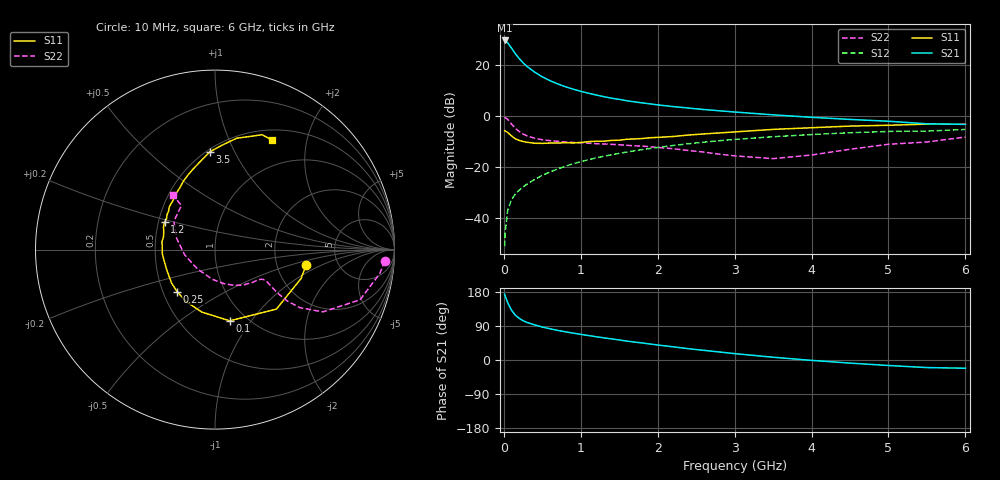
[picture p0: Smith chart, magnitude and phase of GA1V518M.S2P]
! Infineon Technologies  Discrete & RF Semiconductors
! BF775
! Si NPN RF Bipolar Junction Transistor in SOT23
! VCE = 1.5 V  IC = 18 mA
! Common Emitter S-Parameters:  May  1996
# GHz  S  MA  R  50
!  f  S11  S21  S12  S22
! GHz  MAG  ANG  MAG  ANG  MAG  ANG  MAG  ANG
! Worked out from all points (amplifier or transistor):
!   36 points, 10 MHz to 6 GHz, reference 50 ohm
!   highest |S21| = 29.6 dB at 10 MHz (marker M1)
!   |S21| within 3 dB of that: start of sweep to 99.22 MHz
!   unconditionally stable (mu >= 1): 326.7 MHz to end of sweep
!   at 250 MHz: K = 0.91, MSG = 24.3 dB, |S12| = -27.8 dB
!   at 1.4 GHz: K = 1.17, MAG = 8.6 dB, |S12| = -15.2 dB
!   at 6 GHz: K = 1.02, MAG = 0.2 dB, |S12| = -5.3 dB
!   S11 on the Smith chart (normalised r, x): 10 MHz: 2.94, -0.69; 100 MHz: 0.84, -0.79; 250 MHz: 0.59, -0.31; 1.2 GHz: 0.54, +0.18; 3.5 GHz: 0.52, +0.80; 6 GHz: 0.63, +1.45
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0.01  0.5145 -9.6  30.2 173.7  0.0028 81.6  0.9471 -3.9
0.02  0.5058 -18.6  29.73 167.5  0.0056 81.5  0.9282 -8.2
0.05  0.4765 -44.1  27.17 151.2  0.014 73.2  0.8551 -19.1
0.1  0.4052 -78.3  21.3 131.3  0.023 65.9  0.6941 -30.0
0.15  0.3557 -102.0  16.54 118.1  0.0296 62.8  0.5721 -34.4
0.2  0.3312 -119.1  13.34 109.9  0.0351 62.8  0.495 -35.4
0.25  0.3153 -132.2  11 103.7  0.0406 63.7  0.4423 -35.0
0.3  0.3053 -142.5  9.382 99.2  0.0459 64.8  0.4079 -34.3
0.4  0.2917 -157.1  7.23 92.6  0.0568 66.5  0.3666 -32.9
0.5  0.2901 -167.3  5.834 87.0  0.0683 67.7  0.3421 -31.8
0.6  0.2943 -175.6  4.913 82.4  0.0799 67.8  0.3279 -31.5
0.7  0.2944 177.4  4.25 78.1  0.0915 68.1  0.3182 -31.7
0.8  0.2985 171.5  3.739 74.5  0.1035 67.1  0.3091 -32.3
0.9  0.2955 165.8  3.352 70.9  0.1156 66.7  0.303 -33.1
1.1  0.3135 156.2  2.789 64.5  0.1385 65.4  0.2922 -35.9
1.2  0.3192 151.5  2.577 61.4  0.1505 64.4  0.286 -37.4
1.6  0.3491 136.7  1.987 49.8  0.1964 59.8  0.2657 -45.3
2.2  0.3956 119.8  1.526 34.8  0.2635 52.3  0.2276 -61.2
3.5  0.5453 93.1  1.052 7.3  0.3916 34.0  0.1456 -132.7
4.5  0.6326 78.9  0.855 -8.2  0.4684 19.9  0.2224 163.7
5.5  0.6915 67.7  0.701 -20.0  0.5051 5.5  0.3088 127.3
6  0.6886 62.6  0.683 -21.7  0.5439 1.4  0.3859 127.7
